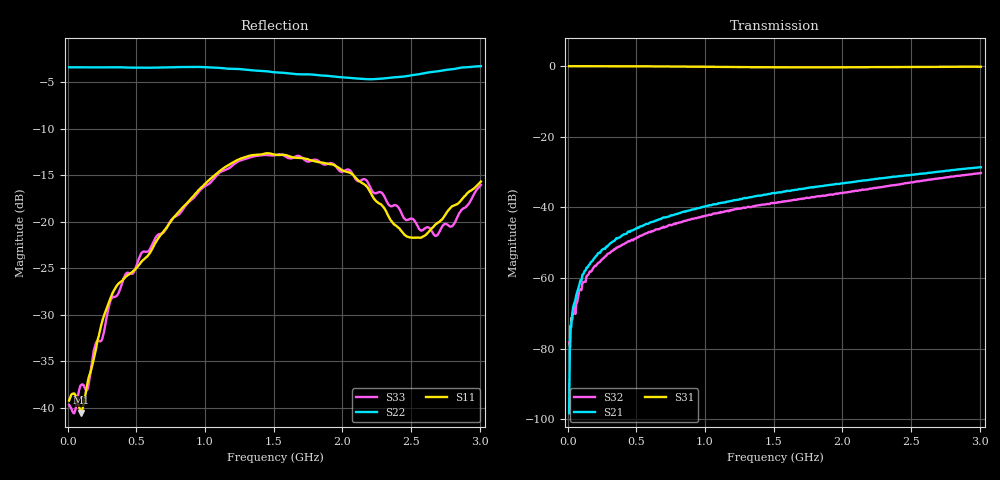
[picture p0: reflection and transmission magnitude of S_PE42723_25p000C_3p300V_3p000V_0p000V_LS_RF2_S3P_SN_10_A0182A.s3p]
! Device ID: PE42723
! File Path: z:\PE42723\Char_75Ohm_20150820\25p000C\3p300\LS_RF2\PE42723_25p000C_3p300V_3p000V_0p000V_LS_RF2_S3P_SN_10_A0182A.s3p
! Serial: 10
! Lot: A0182A
! Temp: 25.000C
! VDD: 3.300
! VSS: 0.000
! Control_Hi: 3.000
! Control_Lo: 0.000
! Logic State: LS_RF2
! Port 1: RFC
! Port 2: RF1
! Port 3: RF2
! ThroughPath:1-3
! IDD: 0.0001155361
! ISS: -1.769e-007
! Comment:
#  Hz  S  RI  R  75
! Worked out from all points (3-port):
!   401 points, 10 MHz to 3.01 GHz, reference 75 ohm
!   strongest paths, dB at 10 MHz, 760 MHz, 1.51 GHz, 2.26 GHz, 3.01 GHz:
!     S31: -0.1, -0.2, -0.4, -0.3, -0.2
!     S21: -98.3, -42.3, -36.1, -31.9, -28.7
!     S32: -78.2, -45.0, -38.7, -34.4, -30.3
!   lowest |S11| = -40.5 dB at 100 MHz (marker M1), VSWR 1.02, Z = 76.3 - j0.676 ohm
!   |S11| at or under -10 dB: start of sweep to end of sweep
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1e7  0.011 -0.000245  4.03e-05 8.5e-05  0.9904 -0.00293
     8.2e-07 1.21e-05  -0.6771 0.00165  3.31e-05 1.73e-05
     0.9903 -0.00292  2.39e-05 0.000121  0.0104 0.000198
4.75e7  0.0119 -0.0009  1.96e-05 0.000505  0.9907 -0.0133
        6.95e-05 0.000432  -0.6767 0.00912  -1.62e-06 0.000355
        0.9907 -0.0132  8.58e-05 0.000413  0.00901 -0.00252
1e8  0.0083 -0.00443  -7.7e-05 0.000946  0.9905 -0.0286
     -1.3e-05 0.00092  -0.6766 0.0186  -8.83e-06 0.000769
     0.9906 -0.0287  4.56e-06 0.000672  0.0113 -0.00705
3.625e8  0.0127 -0.0442  -1.07e-05 0.00367  0.9851 -0.1042
         -1.06e-05 0.00362  -0.6751 0.0576  0.000232 0.00262
         0.983 -0.1052  9.42e-05 0.00269  0.00883 -0.0395
1.0975e9  -0.0516 -0.1776  0.00102 0.0113  0.9241 -0.2953
          0.00102 0.0114  -0.6628 0.1146  0.000507 0.00823
          0.9237 -0.2953  0.000592 0.00832  -0.0526 -0.1735
1.51e9  -0.0721 -0.218  0.00192 0.0158  0.8769 -0.3823
        0.00189 0.0156  -0.6157 0.1592  0.000889 0.0114
        0.8769 -0.3822  0.00105 0.0115  -0.0714 -0.2165
2.065e9  -0.0798 -0.1637  0.00396 0.0223  0.8179 -0.4972
         0.00394 0.0223  -0.5225 0.2797  0.00159 0.0165
         0.8183 -0.4972  0.00147 0.0165  -0.0653 -0.1741
2.5e9  -0.0513 -0.0645  0.00639 0.0278  0.7606 -0.5958
       0.00649 0.028  -0.4432 0.4223  0.00272 0.0221
       0.7626 -0.5927  0.00252 0.0222  -0.0191 -0.1024
2.6875e9  -0.0782 -0.0586  0.00799 0.0307  0.7265 -0.6463
          0.00833 0.0305  -0.435 0.4737  0.00378 0.0249
          0.7274 -0.643  0.00349 0.0251  -0.025 -0.0805
3.01e9  -0.1358 -0.0932  0.0116 0.0351  0.6481 -0.7218
        0.0117 0.0349  -0.4465 0.5213  0.00703 0.0296
        0.6496 -0.7226  0.00704 0.0297  -0.1045 -0.118
